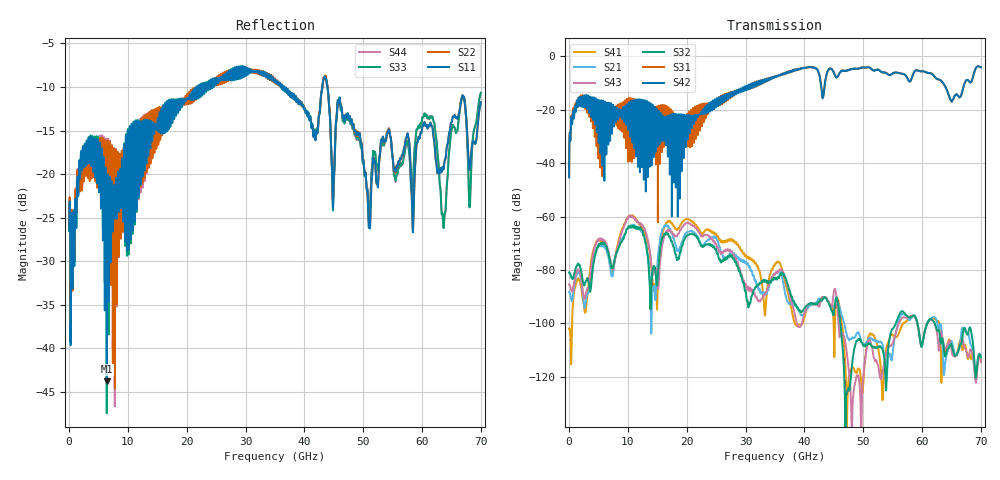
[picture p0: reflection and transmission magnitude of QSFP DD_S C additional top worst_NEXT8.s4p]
! AWR Design Environment (8415) Fri Dec 21 09:14:31 2018
! Document = 'CHANNEL TEST'
! nPorts: 4, nXvals: 7001
# HZ S DB R 50
!Freq DBS11 AngS11 DBS12 AngS12 DBS13 AngS13 DBS14 AngS14
!	DBS21 AngS21 DBS22 AngS22 DBS23 AngS23 DBS24 AngS24
!	DBS31 AngS31 DBS32 AngS32 DBS33 AngS33 DBS34 AngS34
!	DBS41 AngS41 DBS42 AngS42 DBS43 AngS43 DBS44 AngS44
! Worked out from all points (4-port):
!   7000 points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, 10 MHz to 70 GHz, reference 50 ohm
!   strongest paths, dB at 10 MHz, 17.51 GHz, 35.01 GHz, 52.51 GHz, 70 GHz:
!     S42: -45.3, -29.9, -7.6, -5.0, -4.0
!     S31: -45.1, -23.1, -7.6, -5.0, -4.0
!     S32: -80.9, -69.4, -83.5, -108.7, -112.7
!     S43: -85.4, -65.8, -81.6, -115.5, -114.5
!     S21: -88.2, -66.2, -81.5, -106.7, -112.2
!     S41: -101.9, -62.4, -77.8, -109.0, -114.0
!   lowest |S11| = -43.8 dB at 6.41 GHz (marker M1), VSWR 1.01, Z = 50.5 - j0.428 ohm
!   |S11| at or under -10 dB: start of sweep to 21.78 GHz; 36.52 GHz to 43.04 GHz (6.515 GHz wide, 16.4 % of centre); 43.91 GHz to end of sweep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
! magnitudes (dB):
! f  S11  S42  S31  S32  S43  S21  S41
! 10 MHz  -26.5  -45.3  -45.1  -80.9  -85.4  -88.2  -101.9
! 1.64 GHz  -20.2  -15.4  -15.4  -78.1  -80.2  -81.1  -83.7
! 6.41 GHz  -43.8  -20.0  -18.7  -71.5  -70.6  -72.8  -71.6
! 20.23 GHz  -11.3  -25.7  -32.5  -66.8  -62.2  -65.6  -60.9
! 30.78 GHz  -8.1  -11.6  -11.9  -92.6  -86.6  -79.3  -75.7
! 63.65 GHz  -19.4  -10.2  -10.2  -108.4  -107.4  -117.8  -109.4
! 70 GHz  -11.8  -4.0  -4.0  -112.7  -114.5  -112.2  -114.0
